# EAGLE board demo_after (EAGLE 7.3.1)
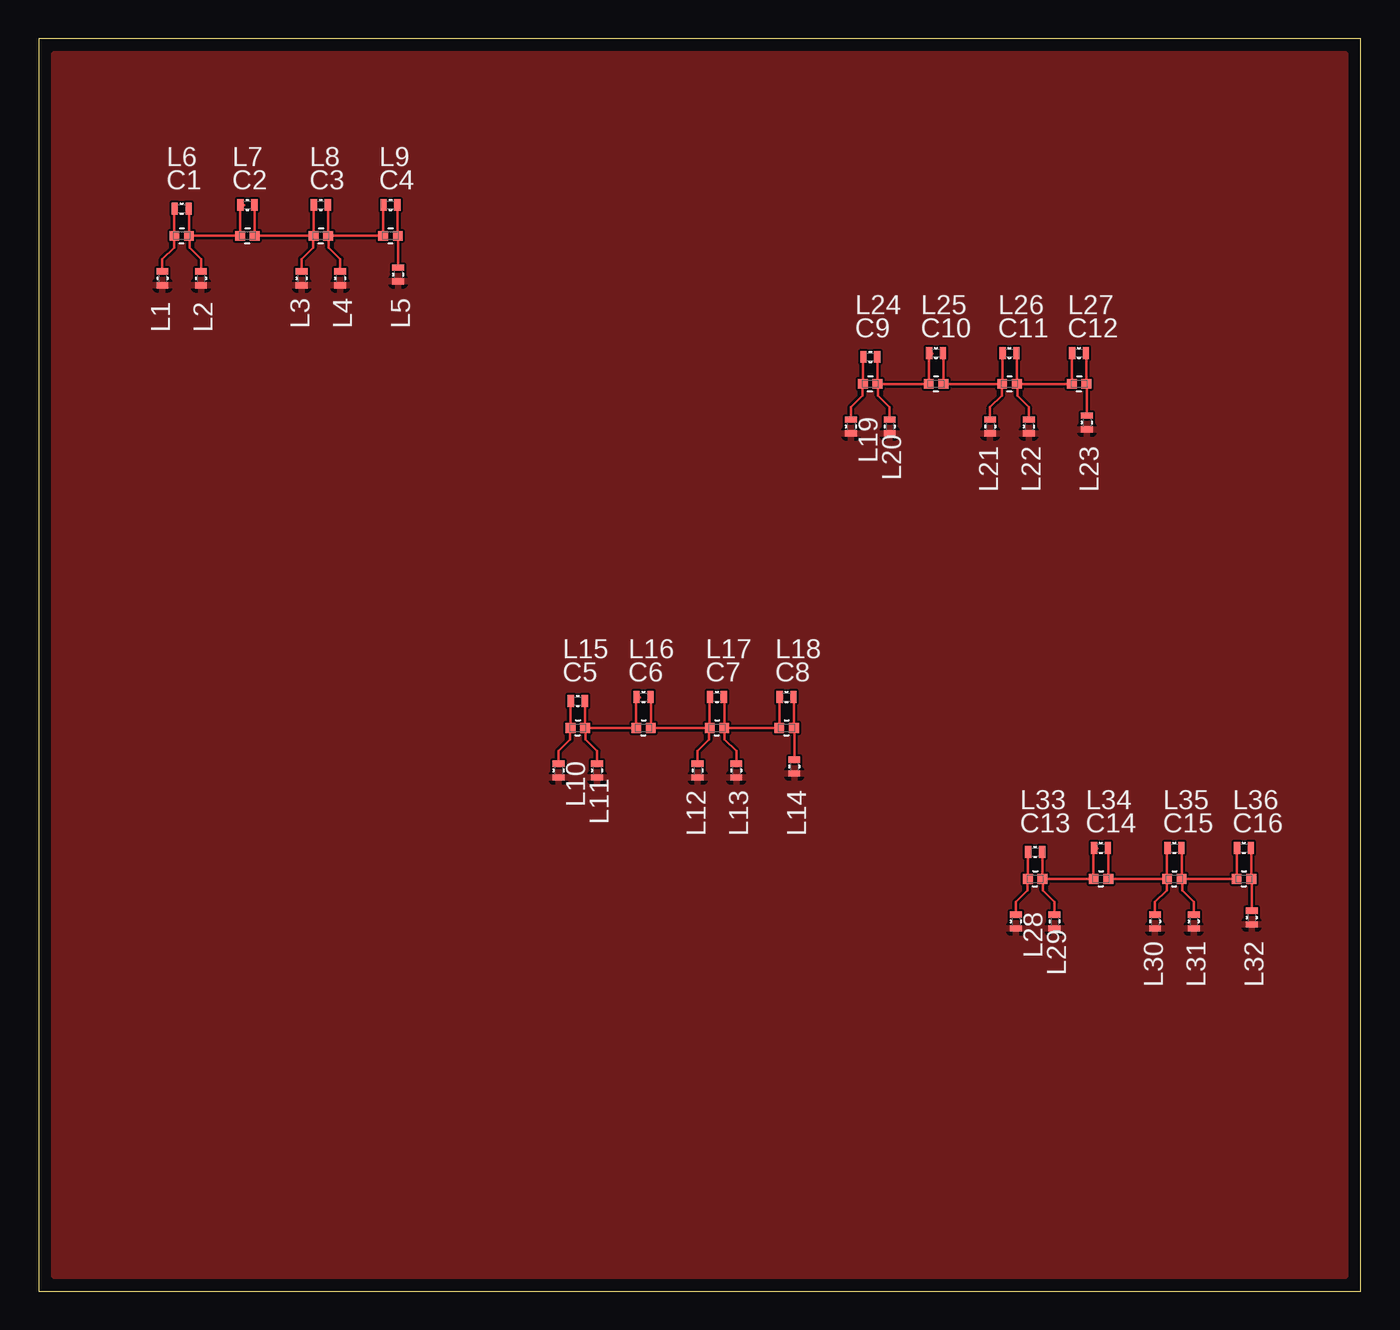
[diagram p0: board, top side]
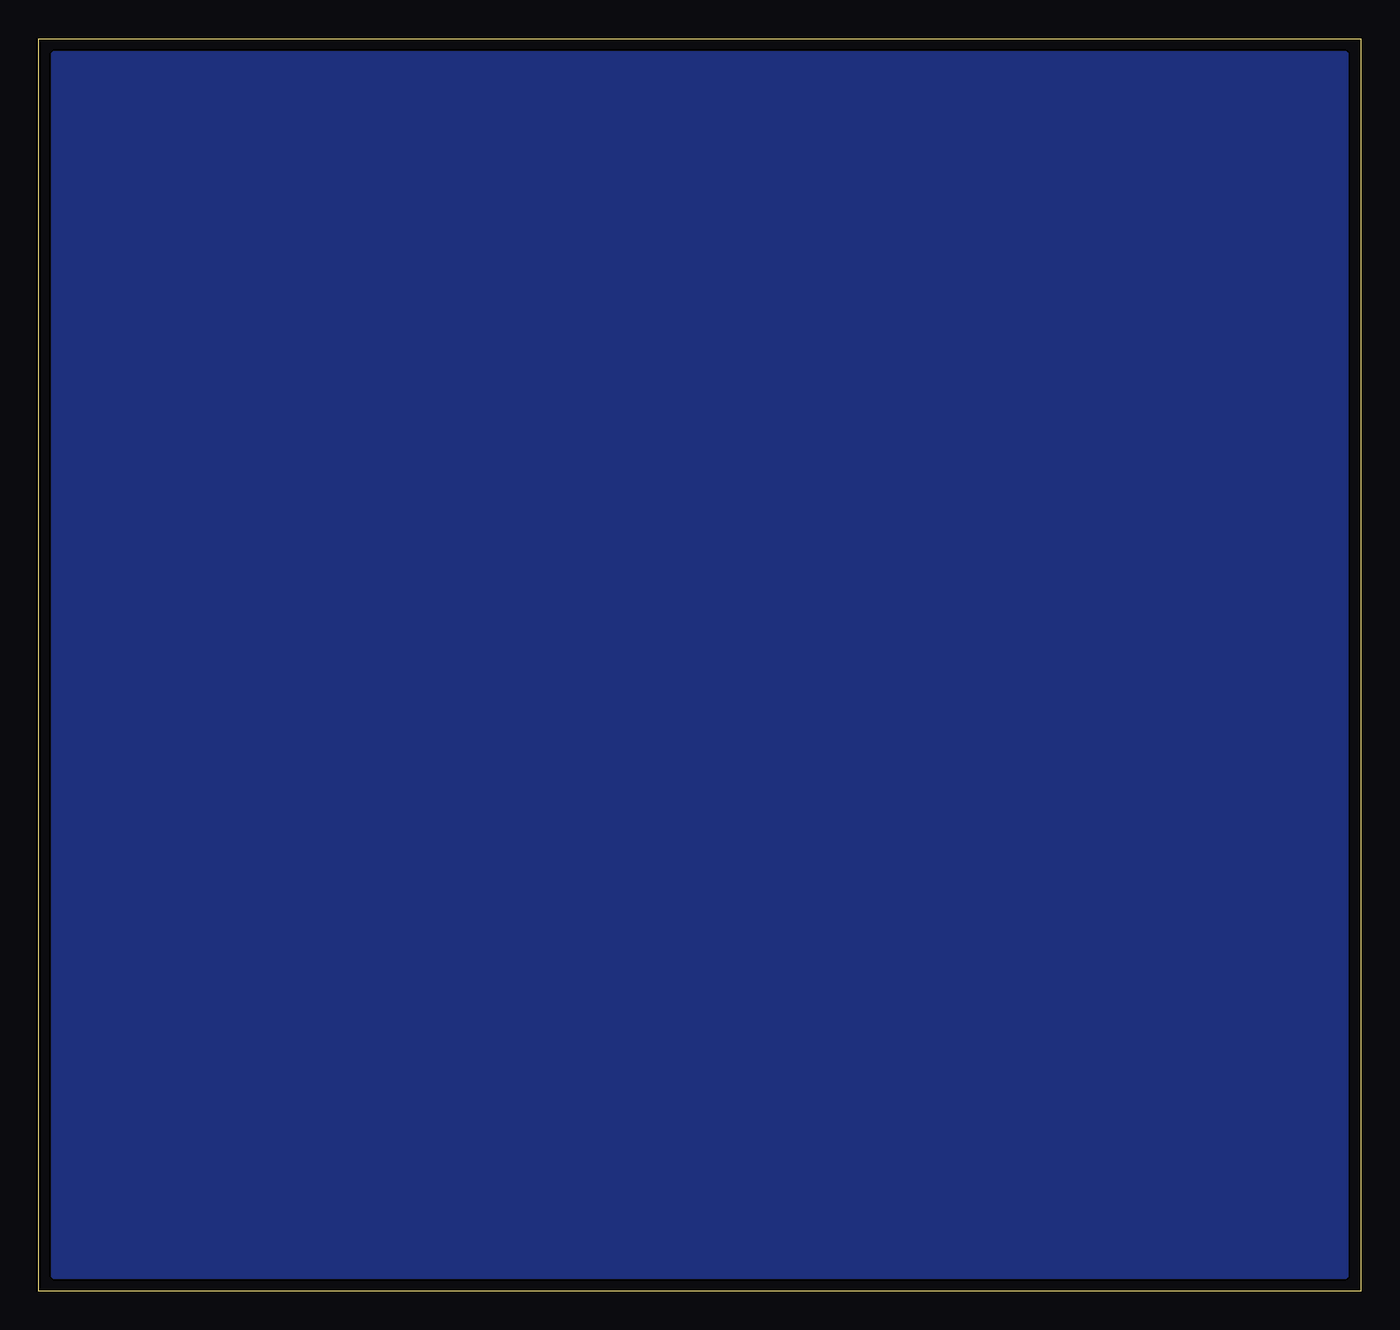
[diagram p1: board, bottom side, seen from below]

Size 85.5 x 81 mm. Coordinates in mm from the lower left corner, seen from the top.
Outline: 0,0 85.5,0 85.5,81 0,81 0,0
Copper layers (1*16): Top 0.0178mm / dielectric 59mil / Bottom 0.0178mm
Design rules "SSC-EAGLE-2Lyr_v1.0.0.3 *": minimum track width 6mil, minimum drill 14mil, track to track 6mil, track to pad 6mil, pad to pad 6mil, via to via 6mil, smd to smd 6mil, copper to edge 20mil, drill to drill 16mil, minimum pad ring 8mil, minimum via ring 8mil, stop-mask expansion 3mil, vias tented up to drill 0mil, thermal gap 10mil

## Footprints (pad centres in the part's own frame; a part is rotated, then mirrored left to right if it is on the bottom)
LTDB_PASSIVES_C0402 = smd 0.635 x 0.635: 1 -0.472,0; 2 0.472,0
LTDB_PASSIVES_R0402 = smd 0.406 x 0.762: 1 -0.447,0; 2 0.447,0

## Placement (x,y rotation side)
C1  [LTDB_PASSIVES_C0402]  9.25,68.25 0 top
C2  [LTDB_PASSIVES_C0402]  13.5,68.25 0 top
C3  [LTDB_PASSIVES_C0402]  18.25,68.25 0 top
C4  [LTDB_PASSIVES_C0402]  22.75,68.25 0 top
C5  [LTDB_PASSIVES_C0402]  34.86,36.42 0 top
C6  [LTDB_PASSIVES_C0402]  39.11,36.42 0 top
C7  [LTDB_PASSIVES_C0402]  43.86,36.42 0 top
C8  [LTDB_PASSIVES_C0402]  48.36,36.42 0 top
C9  [LTDB_PASSIVES_C0402]  53.78,58.67 0 top
C10  [LTDB_PASSIVES_C0402]  58.03,58.67 0 top
C11  [LTDB_PASSIVES_C0402]  62.78,58.67 0 top
C12  [LTDB_PASSIVES_C0402]  67.28,58.67 0 top
C13  [LTDB_PASSIVES_C0402]  64.44,26.66 0 top
C14  [LTDB_PASSIVES_C0402]  68.69,26.66 0 top
C15  [LTDB_PASSIVES_C0402]  73.44,26.66 0 top
C16  [LTDB_PASSIVES_C0402]  77.94,26.66 0 top
L1  [LTDB_PASSIVES_R0402]  8,65.5 270 top
L2  [LTDB_PASSIVES_R0402]  10.5,65.5 270 top
L3  [LTDB_PASSIVES_R0402]  17,65.5 270 top
L4  [LTDB_PASSIVES_R0402]  19.5,65.5 270 top
L5  [LTDB_PASSIVES_R0402]  23.25,65.75 270 top
L6  [LTDB_PASSIVES_R0402]  9.25,70 0 top
L7  [LTDB_PASSIVES_R0402]  13.5,70.25 0 top
L8  [LTDB_PASSIVES_R0402]  18.25,70.25 0 top
L9  [LTDB_PASSIVES_R0402]  22.75,70.25 0 top
L10  [LTDB_PASSIVES_R0402]  33.61,33.67 270 top
L11  [LTDB_PASSIVES_R0402]  36.11,33.67 270 top
L12  [LTDB_PASSIVES_R0402]  42.61,33.67 270 top
L13  [LTDB_PASSIVES_R0402]  45.11,33.67 270 top
L14  [LTDB_PASSIVES_R0402]  48.86,33.92 270 top
L15  [LTDB_PASSIVES_R0402]  34.86,38.17 0 top
L16  [LTDB_PASSIVES_R0402]  39.11,38.42 0 top
L17  [LTDB_PASSIVES_R0402]  43.86,38.42 0 top
L18  [LTDB_PASSIVES_R0402]  48.36,38.42 0 top
L19  [LTDB_PASSIVES_R0402]  52.53,55.92 270 top
L20  [LTDB_PASSIVES_R0402]  55.03,55.92 270 top
L21  [LTDB_PASSIVES_R0402]  61.53,55.92 270 top
L22  [LTDB_PASSIVES_R0402]  64.03,55.92 270 top
L23  [LTDB_PASSIVES_R0402]  67.78,56.17 270 top
L24  [LTDB_PASSIVES_R0402]  53.78,60.42 0 top
L25  [LTDB_PASSIVES_R0402]  58.03,60.67 0 top
L26  [LTDB_PASSIVES_R0402]  62.78,60.67 0 top
L27  [LTDB_PASSIVES_R0402]  67.28,60.67 0 top
L28  [LTDB_PASSIVES_R0402]  63.19,23.91 270 top
L29  [LTDB_PASSIVES_R0402]  65.69,23.91 270 top
L30  [LTDB_PASSIVES_R0402]  72.19,23.91 270 top
L31  [LTDB_PASSIVES_R0402]  74.69,23.91 270 top
L32  [LTDB_PASSIVES_R0402]  78.44,24.16 270 top
L33  [LTDB_PASSIVES_R0402]  64.44,28.41 0 top
L34  [LTDB_PASSIVES_R0402]  68.69,28.66 0 top
L35  [LTDB_PASSIVES_R0402]  73.44,28.66 0 top
L36  [LTDB_PASSIVES_R0402]  77.94,28.66 0 top

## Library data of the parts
C1-C16 L1-L36 = vnatest

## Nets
GND: L1.2 L2.2 L3.2 L4.2 L5.2 L10.2 L11.2 L12.2 L13.2 L14.2 L19.2 L20.2 L21.2 L22.2 L23.2 L28.2 L29.2 L30.2 L31.2 L32.2
IN1: C1.1 L1.1 L6.1
IN2: C5.1 L10.1 L15.1
IN3: C9.1 L19.1 L24.1
IN4: C13.1 L28.1 L33.1
N$1: C5.2 C6.1 L11.1 L15.2 L16.1
N$2: C6.2 C7.1 L12.1 L16.2 L17.1
N$3: C7.2 C8.1 L13.1 L17.2 L18.1
N$4: C9.2 C10.1 L20.1 L24.2 L25.1
N$5: C10.2 C11.1 L21.1 L25.2 L26.1
N$6: C11.2 C12.1 L22.1 L26.2 L27.1
N$7: C13.2 C14.1 L29.1 L33.2 L34.1
N$8: C14.2 C15.1 L30.1 L34.2 L35.1
N$9: C15.2 C16.1 L31.1 L35.2 L36.1
N$20: C1.2 C2.1 L2.1 L6.2 L7.1
N$21: C2.2 C3.1 L3.1 L7.2 L8.1
N$22: C3.2 C4.1 L4.1 L8.2 L9.1
OUT1: C4.2 L5.1 L9.2
OUT2: C8.2 L14.1 L18.2
OUT3: C12.2 L23.1 L27.2
OUT4: C16.2 L32.1 L36.2

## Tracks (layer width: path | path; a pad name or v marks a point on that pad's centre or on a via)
GND
  pour Bottom: 1,80 84.5,80 84.5,1 1,1
  pour Top: 1,80 84.5,80 84.5,1 1,1
IN1
  Top 0.152: L1.1 8,66.75 8.75,67.5 8.75,68.22 C1.1 8.78,69.97 L6.1
IN2
  Top 0.152: L10.1 33.61,34.92 34.36,35.67 34.36,36.4 C5.1 34.39,38.15 L15.1
IN3
  Top 0.152: L19.1 52.53,57.17 53.28,57.92 53.28,58.65 C9.1 53.3,60.4 L24.1
IN4
  Top 0.152: L28.1 63.19,25.16 63.94,25.91 63.94,26.63 C13.1 63.97,28.39 L33.1
N$1
  Top 0.152: C5.2 35.34,38.15 L15.2 | L11.1 36.11,34.92 35.36,35.67 35.36,36.4 C5.2 | 38.89,38.4 L16.1 38.64,38.4 C6.1 C5.2
N$2
  Top 0.152: L16.2 39.59,38.4 C6.2 C7.1 | C7.1 43.39,38.4 L17.1 | L12.1 42.61,34.92 43.36,35.67 43.36,36.4 C7.1
N$3
  Top 0.152: C7.2 C8.1 47.89,38.4 L18.1 | C7.2 44.34,38.4 L17.2 | L13.1 45.11,34.92 44.36,35.67 44.36,36.4 C7.2
N$4
  Top 0.152: C9.2 54.25,60.4 L24.2 | L20.1 55.03,57.17 54.28,57.92 54.28,58.65 C9.2 | 57.8,60.65 L25.1 57.55,60.65 C10.1 C9.2
N$5
  Top 0.152: L25.2 58.5,60.65 C10.2 C11.1 | C11.1 62.3,60.65 L26.1 | L21.1 61.53,57.17 62.28,57.92 62.28,58.65 C11.1
N$6
  Top 0.152: C11.2 C12.1 66.81,60.65 L27.1 | C11.2 63.25,60.65 L26.2 | L22.1 64.03,57.17 63.28,57.92 63.28,58.65 C11.2
N$7
  Top 0.152: C13.2 64.91,28.39 L33.2 | L29.1 65.69,25.16 64.94,25.91 64.94,26.63 C13.2 | 68.47,28.64 L34.1 68.22,28.64 C14.1 C13.2
N$8
  Top 0.152: L34.2 69.16,28.64 C14.2 C15.1 | C15.1 72.97,28.64 L35.1 | L30.1 72.19,25.16 72.94,25.91 72.94,26.63 C15.1
N$9
  Top 0.152: C15.2 C16.1 77.47,28.64 L36.1 | C15.2 73.91,28.64 L35.2 | L31.1 74.69,25.16 73.94,25.91 73.94,26.63 C15.2
N$20
  Top 0.152: C1.2 9.72,69.97 L6.2 | L2.1 10.5,66.75 9.75,67.5 9.75,68.22 C1.2 | 13.28,70.22 L7.1 13.03,70.22 C2.1 C1.2
N$21
  Top 0.152: L7.2 13.97,70.22 C2.2 C3.1 | C3.1 17.78,70.22 L8.1 | L3.1 17,66.75 17.75,67.5 17.75,68.22 C3.1
N$22
  Top 0.152: C3.2 C4.1 22.28,70.22 L9.1 | C3.2 18.72,70.22 L8.2 | L4.1 19.5,66.75 18.75,67.5 18.75,68.22 C3.2
OUT1
  Top 0.152: L9.2 23.22,70.22 C4.2 23.25,68.22 L5.1
OUT2
  Top 0.152: L18.2 48.84,38.4 C8.2 48.86,36.4 L14.1
OUT3
  Top 0.152: L27.2 67.75,60.65 C12.2 67.78,58.65 L23.1
OUT4
  Top 0.152: L36.2 78.41,28.64 C16.2 78.44,26.63 L32.1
